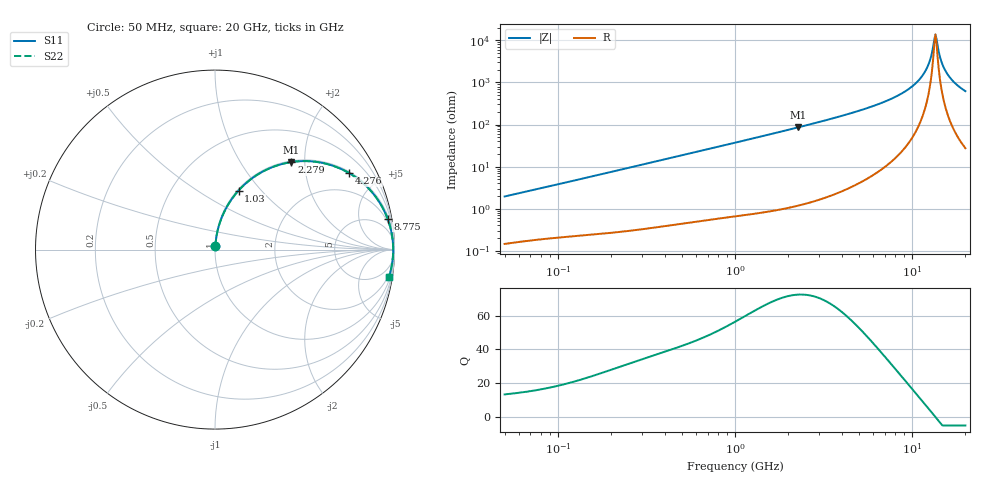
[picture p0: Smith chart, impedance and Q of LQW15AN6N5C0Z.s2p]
!Murata Part Number: LQW15AN6N5C0Z
!These Parameters are Measured in Series Mode Connection
!  o--[Z]--o
!Port1  Port2
!  o-------o
!Freq. Start=50[MHz] Stop=20[GHz], 401[Steps]
# Hz S RI R 50
!Freq.(Hz) S11(Real) S11(Imag) S21(Real) S21(Imag) S12(Real) S12(Imag) S22(Real) S22(Imag)
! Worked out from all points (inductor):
!   401 points, 50 MHz to 20 GHz, reference 50 ohm
!   read as one part in series: L = 6.14 nH near 51.52 MHz
!   highest Q = 72.4 at 2.279 GHz (marker M1), where L = 6 nH
!   self-resonance near 13.55 GHz
!   S11 on the Smith chart (normalised r, x): 50 MHz: 1.00, +0.04; 1.03 GHz: 1.01, +0.76; 2.279 GHz: 1.02, +1.72; 4.276 GHz: 1.06, +3.47; 8.775 GHz: 1, +11; 20 GHz: 2, -12
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5e7  0.00183 0.0194  0.9982 -0.0194  0.9982 -0.0194  0.00183 0.0194
1.364002e8  0.00492 0.051  0.9951 -0.051  0.9951 -0.051  0.00492 0.051
3.721004e8  0.0223 0.1348  0.9777 -0.1348  0.9777 -0.1348  0.0223 0.1348
1e9  0.1245 0.3214  0.8755 -0.3214  0.8755 -0.3214  0.1245 0.3214
1.030411e9  0.131 0.3287  0.869 -0.3287  0.869 -0.3287  0.131 0.3287
2.279204e9  0.4254 0.4875  0.5746 -0.4875  0.5746 -0.4875  0.4254 0.4875
2.728004e9  0.5195 0.4927  0.4805 -0.4927  0.4805 -0.4927  0.5195 0.4927
4.275624e9  0.7474 0.4262  0.2526 -0.4262  0.2526 -0.4262  0.7474 0.4262
7.442007e9  0.9318 0.2373  0.0682 -0.2373  0.0682 -0.2373  0.9318 0.2373
8.774992e9  0.9614 0.1727  0.0386 -0.1727  0.0386 -0.1727  0.9614 0.1727
1.034674e10  0.9809 0.1073  0.0191 -0.1073  0.0191 -0.1073  0.9809 0.1073
1.166392e10  0.9891 0.0597  0.0109 -0.0597  0.0109 -0.0597  0.9891 0.0597
1.238412e10  0.9914 0.0359  0.00856 -0.0359  0.00856 -0.0359  0.9914 0.0359
1.276073e10  0.9922 0.0239  0.00782 -0.0239  0.00782 -0.0239  0.9922 0.0239
1.314879e10  0.9926 0.012  0.00737 -0.012  0.00737 -0.012  0.9926 0.012
1.354865e10  0.9928 0.000106  0.00721 -0.000106  0.00721 -0.000106  0.9928 0.000106
1.396067e10  0.9927 -0.0118  0.00733 0.0118  0.00733 0.0118  0.9927 -0.0118
1.438523e10  0.9923 -0.0237  0.00775 0.0237  0.00775 0.0237  0.9923 -0.0237
1.482269e10  0.9916 -0.0357  0.00845 0.0357  0.00845 0.0357  0.9916 -0.0357
1.573793e10  0.9893 -0.0595  0.0107 0.0595  0.0107 0.0595  0.9893 -0.0595
1.747767e10  0.9825 -0.1012  0.0175 0.1012  0.0175 0.1012  0.9825 -0.1012
2e10  0.9682 -0.1548  0.0318 0.1548  0.0318 0.1548  0.9682 -0.1548
